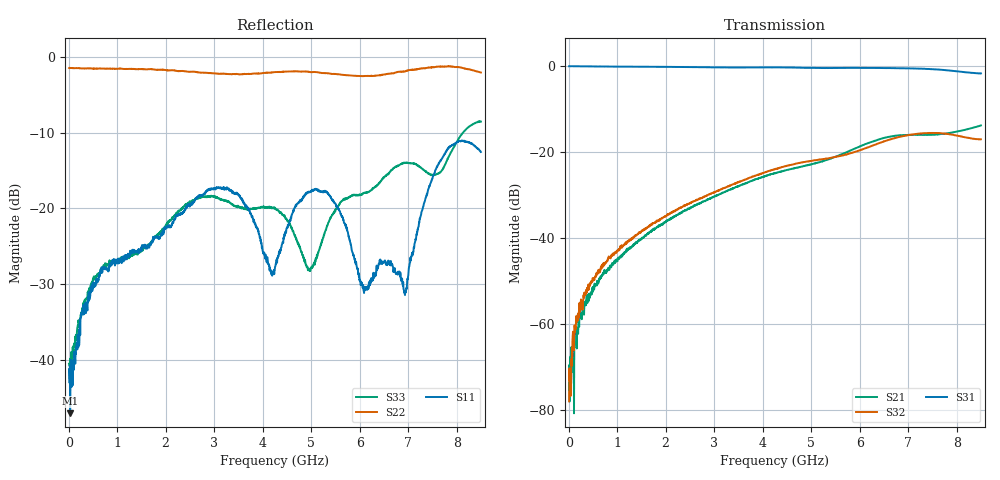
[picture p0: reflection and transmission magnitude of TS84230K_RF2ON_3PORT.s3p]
! Created with skrf (http://scikit-rf.org).
# Hz S RI R 50.0
!freq ReS11 ImS11 ReS12 ImS12 ReS13 ImS13
! ReS21 ImS21 ReS22 ImS22 ReS23 ImS23
! ReS31 ImS31 ReS32 ImS32 ReS33 ImS33
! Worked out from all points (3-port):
!   1601 points, 10 MHz to 8.5 GHz, reference 50 ohm
!   strongest paths, dB at 10 MHz, 2.132 GHz, 4.255 GHz, 6.378 GHz, 8.5 GHz:
!     S31: -0.1, -0.3, -0.4, -0.5, -1.8
!     S32: -78.0, -34.0, -24.1, -18.1, -17.1
!     S21: -75.5, -35.3, -24.9, -17.2, -13.9
!   lowest |S11| = -47.1 dB at 31.23 MHz (marker M1), VSWR 1.01, Z = 50.4 - j0.127 ohm
!   |S11| at or under -10 dB: start of sweep to end of sweep
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1e7  0.00808 -0.00309  -4.84e-05 0.000103  0.9884 -0.00523
     0.000167 -5.36e-06  -0.8473 0.00452  1.28e-05 3.77e-05
     0.9879 -0.00497  5.6e-05 0.000113  0.00936 -0.000948
3.1225e7  0.00423 -0.00126  -0.000129 0.000289  0.9885 -0.0121
          0.000109 0.000293  -0.8478 0.00933  2.92e-05 0.000225
          0.9883 -0.012  0.000208 0.000143  0.00977 -0.00279
2.275562e8  0.00608 -0.0145  0.000175 0.000992  0.9828 -0.0812
            -0.000228 0.00115  -0.842 0.0779  0.000137 0.00147
            0.9825 -0.0807  -8.77e-05 0.00137  0.00923 -0.0157
8.908375e8  -0.0127 -0.0404  -0.000527 0.0047  0.9306 -0.3056
            -0.000879 0.00482  -0.781 0.3008  -6.51e-05 0.0062
            0.931 -0.3052  2.18e-05 0.00614  -0.00683 -0.0437
3.082319e9  -0.1036 -0.0904  0.00052 0.0314  0.4461 -0.8477
            0.000371 0.0317  -0.1984 0.7501  0.0158 0.0315
            0.4464 -0.8476  0.0159 0.0313  -0.0974 -0.065
4.255e9  -0.0056 0.0405  0.021 0.0523  0.0627 -0.9565
         0.0211 0.0525  0.4021 0.6878  0.0509 0.0369
         0.064 -0.9561  0.0508 0.0368  -0.0236 -0.0983
5.109306e9  0.1213 0.0569  0.043 0.0605  -0.2394 -0.9136
            0.0431 0.0607  0.6601 0.4452  0.0784 0.0176
            -0.2376 -0.9135  0.0784 0.0177  0.0437 -0.0155
6.934656e9  0.0168 0.0208  0.1555 0.0194  -0.7896 -0.4997
            0.1554 0.0197  0.6503 -0.4785  0.1251 -0.0892
            -0.7884 -0.5006  0.1255 -0.0891  -0.1252 -0.1551
7.624469e9  0.1132 -0.1597  0.1573 -0.0268  -0.8829 -0.1971
            0.1575 -0.0265  0.4335 -0.7492  0.0655 -0.1519
            -0.8832 -0.1983  0.0654 -0.1517  -0.0366 -0.1665
8.5e9  -0.0776 -0.2233  0.1833 -0.0869  -0.8012 0.1526
       0.1834 -0.0864  0.2175 -0.7613  -0.00389 -0.14
       -0.801 0.1491  -0.00321 -0.14  0.146 -0.3452
